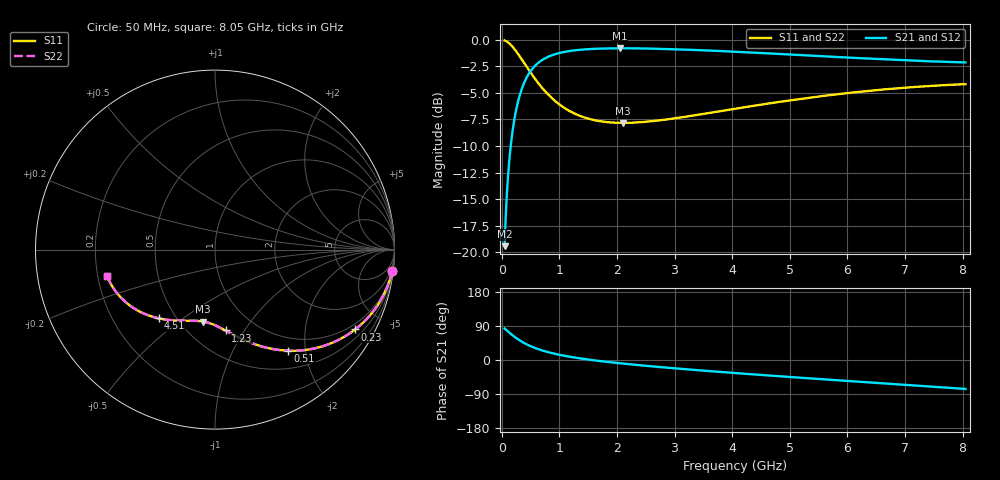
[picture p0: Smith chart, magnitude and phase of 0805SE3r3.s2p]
! AVX Thin Film Operation		Date: August 2001
! Description: Accu-P® Series, Thin Film, SMD, RF Capacitor
! Part Number: 08051J3R3ABT
! 50 MHz  -  8.05 GHz
! Serial Measurements
# mhz S db R 50
!	S11		S21		S12		S22
!	dB	Phase	dB	Phase	dB	Phase	dB	Phase
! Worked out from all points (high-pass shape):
!   401 points, 50 MHz to 8.05 GHz, reference 50 ohm
!   highest |S21| = -0.79 dB at 2.05 GHz (marker M1); lowest = -19.4 dB at 50 MHz (marker M2)
!   |S21| within 3 dB of the highest: 410.3 MHz to end of sweep
!   lowest |S11| = -7.8 dB at 2.11 GHz (marker M3), VSWR 2.37, Z = 32.1 - j30.9 ohm
!   |S11| at or under -10 dB: nowhere
!   |S22| runs from -7.8 to 0.0 dB; largest |S21 - S12| = 0
!   S11 on the Smith chart (normalised r, x): 50 MHz: 1, -16; 230 MHz: 0.78, -3.62; 510 MHz: 0.77, -1.69; 1.23 GHz: 0.73, -0.83; 4.51 GHz: 0.40, -0.41; 8.05 GHz: 0.24, -0.11
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50  -0.05 -6.9  -19.44 83.1  -19.44 83.1  -0.05 -6.9
70  -0.10 -9.7  -16.58 80.3  -16.58 80.3  -0.10 -9.7
110  -0.24 -15.0  -12.80 75.0  -12.80 75.0  -0.24 -15.0
150  -0.42 -20.2  -10.32 69.8  -10.32 69.8  -0.42 -20.2
190  -0.66 -25.1  -8.52 64.9  -8.52 64.9  -0.66 -25.1
230  -0.93 -29.7  -7.17 60.3  -7.17 60.3  -0.93 -29.7
350  -1.86 -41.8  -4.59 48.2  -4.59 48.2  -1.86 -41.8
510  -3.15 -54.1  -2.88 35.9  -2.88 35.9  -3.15 -54.1
650  -4.18 -62.2  -2.09 27.7  -2.09 27.7  -4.18 -62.2
810  -5.17 -69.5  -1.58 20.5  -1.58 20.5  -5.17 -69.5
1010  -6.12 -76.5  -1.22 13.5  -1.22 13.5  -6.12 -76.5
1230  -6.85 -82.6  -1.01 7.3  -1.01 7.3  -6.85 -82.6
1390  -7.23 -86.3  -0.92 3.6  -0.92 3.6  -7.23 -86.4
2050  -7.82 -98.5  -0.79 -8.6  -0.79 -8.6  -7.82 -98.6
2110  -7.82 -99.5  -0.79 -9.6  -0.79 -9.6  -7.82 -99.5
2730  -7.59 -108.3  -0.84 -18.4  -0.84 -18.4  -7.59 -108.4
3370  -7.09 -116.4  -0.95 -26.5  -0.95 -26.5  -7.09 -116.4
4050  -6.49 -124.3  -1.11 -34.4  -1.11 -34.4  -6.49 -124.4
4510  -6.09 -129.4  -1.23 -39.5  -1.23 -39.5  -6.09 -129.5
5390  -5.41 -138.8  -1.49 -48.9  -1.49 -48.9  -5.41 -138.9
6730  -4.62 -152.6  -1.85 -62.8  -1.85 -62.8  -4.62 -152.6
8050  -4.17 -166.2  -2.12 -76.3  -2.12 -76.3  -4.17 -166.2
